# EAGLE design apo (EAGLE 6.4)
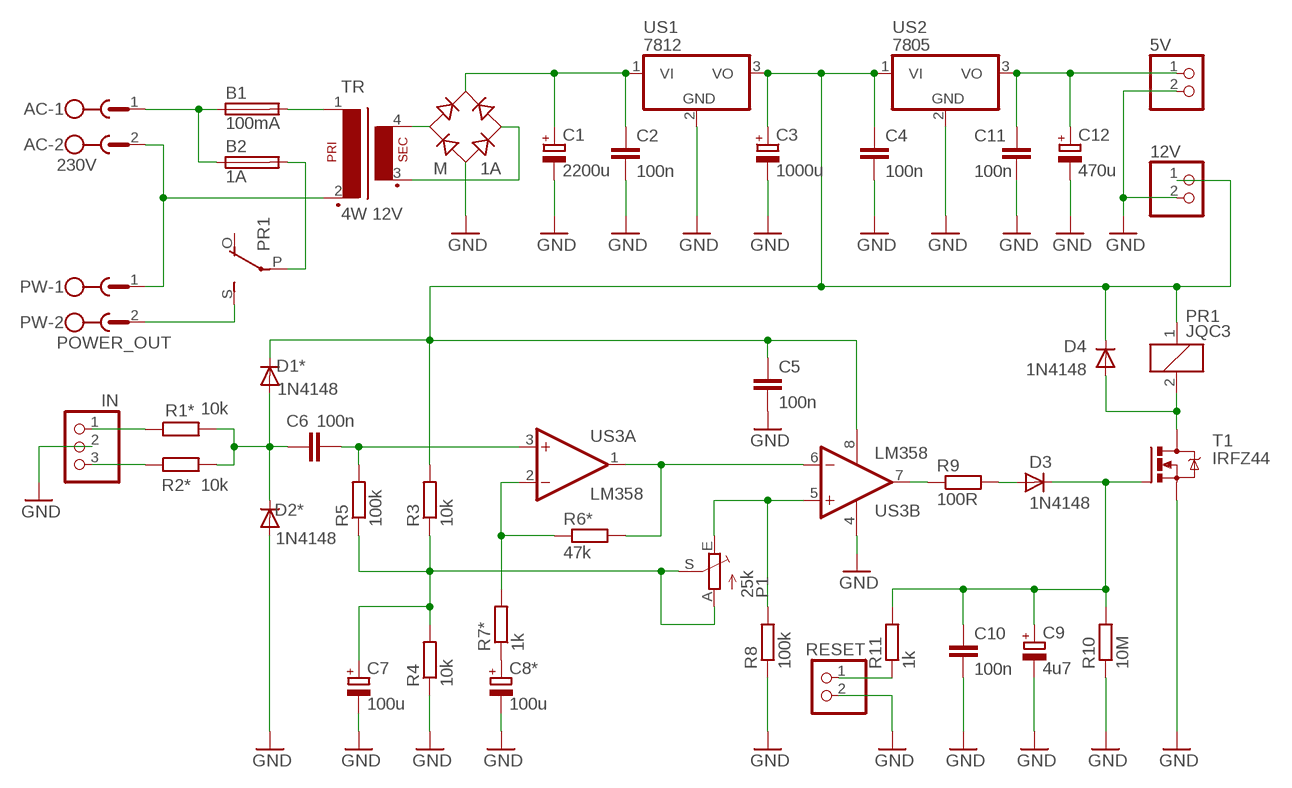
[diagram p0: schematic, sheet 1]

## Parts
5V  PINHD-1X2  [1X02]
12V  PINHD-1X2  [1X02]
AC  230V  MSTBV2  [MSTBV2]
B1  100mA  SH22,5A  [SH22,5A]
B2  1A  SH22,5A  [SH22,5A]
C1  2200u  CPOL-EUE5-13  [E5-13]
C2  100n  C-EU050-025X075  [C050-025X075]
C3  1000u  CPOL-EUE5-10.5  [E5-10,5]
C4  100n  C-EU050-025X075  [C050-025X075]
C5  100n  C-EU050-025X075  [C050-025X075]
C6  100n  C-EU050-025X075  [C050-025X075]
C7  100u  CPOL-EUE2.5-7  [E2,5-7]
C8*  100u  CPOL-EUE2.5-7  [E2,5-7]
C9  4u7  CPOL-EUE5-8.5  [E5-8,5]
C10  100n  C-EU050-025X075  [C050-025X075]
C11  100n  C-EU050-025X075  [C050-025X075]
C12  470u  CPOL-EUE5-8.5  [E5-8,5]
D1*  1N4148  1N4148DO35-7  [DO35-7]
D2*  1N4148  1N4148DO35-7  [DO35-7]
D3  1N4148  1N4148DO35-7  [DO35-7]
D4  1N4148  1N4148DO35-7  [DO35-7]
IN  PINHD-1X3  [1X03]
M  1A  RB1A  [RB1A]
P1  25k  TRIM_EU-RS3  [RS3]
PR1  JQC3  G5L  [G5LE]
PW  POWER_OUT  MSTBV2  [MSTBV2]
R1*  10k  R-EU_0207/10  [0207/10]
R2*  10k  R-EU_0207/10  [0207/10]
R3  10k  R-EU_0207/10  [0207/10]
R4  10k  R-EU_0207/10  [0207/10]
R5  100k  R-EU_0207/10  [0207/10]
R6*  47k  R-EU_0207/10  [0207/10]
R7*  1k  R-EU_0207/10  [0207/10]
R8  100k  R-EU_0207/10  [0207/10]
R9  100R  R-EU_0207/10  [0207/10]
R10  10M  R-EU_0207/10  [0207/10]
R11  1k  R-EU_0207/10  [0207/10]
RESET  PINHD-1X2  [1X02]
T1  IRFZ44  IRF540  [TO220BV]
TR  4W 12V  VP31  [VP31]
US1  7812  7812TV  [TO220V]
US2  7805  7805TV  [TO220V]
US3  LM358  LM358N  [DIL08]

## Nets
GND: 5V.2 12V.2 C1.- C2.2 C3.- C4.2 C5.2 C7.- C8*.- C9.- C10.2 C11.2 C12.- D2*.A IN.2 M.- R4.1 R8.1 R10.1 RESET.2 T1.S US1.2(GND) US2.2(GND) US3.4(P:V-)
N$1: AC.2 PW.1 TR.2
N$2: AC.1 B1.1 B2.1
N$3: B1.2 TR.1
N$4: M.AC1 TR.4(S4)
N$5: B2.2 PR1.P(2:P)
N$6: PR1.S(2:S) PW.2
N$7: M.AC2 TR.3(S3)
N$8: C1.+ C2.1 M.+ US1.1(VI)
N$9: 12V.1 C3.+ C4.1 C5.1 D1*.C D4.C PR1.1 R3.2 US1.3(VO) US2.1(VI) US3.8(P:V+)
N$10: IN.1 R1*.1
N$11: C6.2 R5.2 US3.3(A:+IN)
N$12: IN.3 R2*.1
N$13: R6*.1 R7*.2 US3.2(A:-IN)
N$14: C6.1 D1*.A D2*.C R1*.2 R2*.2
N$15: C8*.+ R7*.1
N$16: R6*.2 US3.1(A:OUT) US3.6(B:-IN)
N$17: C7.+ P1.A P1.S R3.1 R4.2 R5.1
N$18: D4.A PR1.2 T1.D
N$19: P1.E R8.2 US3.5(B:+IN)
N$21: C9.+ C10.1 D3.C R10.2 R11.2 T1.G
N$22: R9.1 US3.7(B:OUT)
N$23: D3.A R9.2
N$25: R11.1 RESET.1
N$26: 5V.1 C11.1 C12.+ US2.3(VO)
Unconnected: PR1.O(2:O)

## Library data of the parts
5V 12V RESET = pinhead:PINHD-1X2: PIN HEADER
AC PW = con-phoenix-508:MSTBV2: PHOENIX
B1 B2 = fuse:SH22,5A: FUSE HOLDER
C1 C3 C7 C8* C9 C12 = rcl:CPOL-EU: POLARIZED CAPACITOR, European symbol
C2 C4-C6 C10 C11 = rcl:C-EU: CAPACITOR, European symbol
D1* D2* D3 D4 = diode:1N4148: DIODE
IN = pinhead:PINHD-1X3: PIN HEADER
M = rectifier:RB1A: RECTIFIER 1 A
P1 = pot:TRIM_EU-: POTENTIOMETER
PR1 = relay:G5L: RELAY 1 x switch, 10 A/120 V AC, 8 A/30 V ADC, Omron
R1* R2* R3-R5 R6* R7* R8-R11 = rcl:R-EU_: RESISTOR, European symbol
T1 = transistor-power:IRF540: HEXFET Power MOSFET
TR = trafo:VP31: TRANSFORMER 1 primary winding, 1 secondary winding BLOCK
US1 US2 = linear:78*: Positive VOLTAGE REGULATOR Source: http://cache.national.com/ds/LM/LM78L05.pdf http://www.fairchildsemi.com/ds/LM/LM7805.pdf
US3 = linear:LM358: OP AMP also LM158; LM258; LM2904 Source: http://cache.national.com/ds/LM/LM158.pdf

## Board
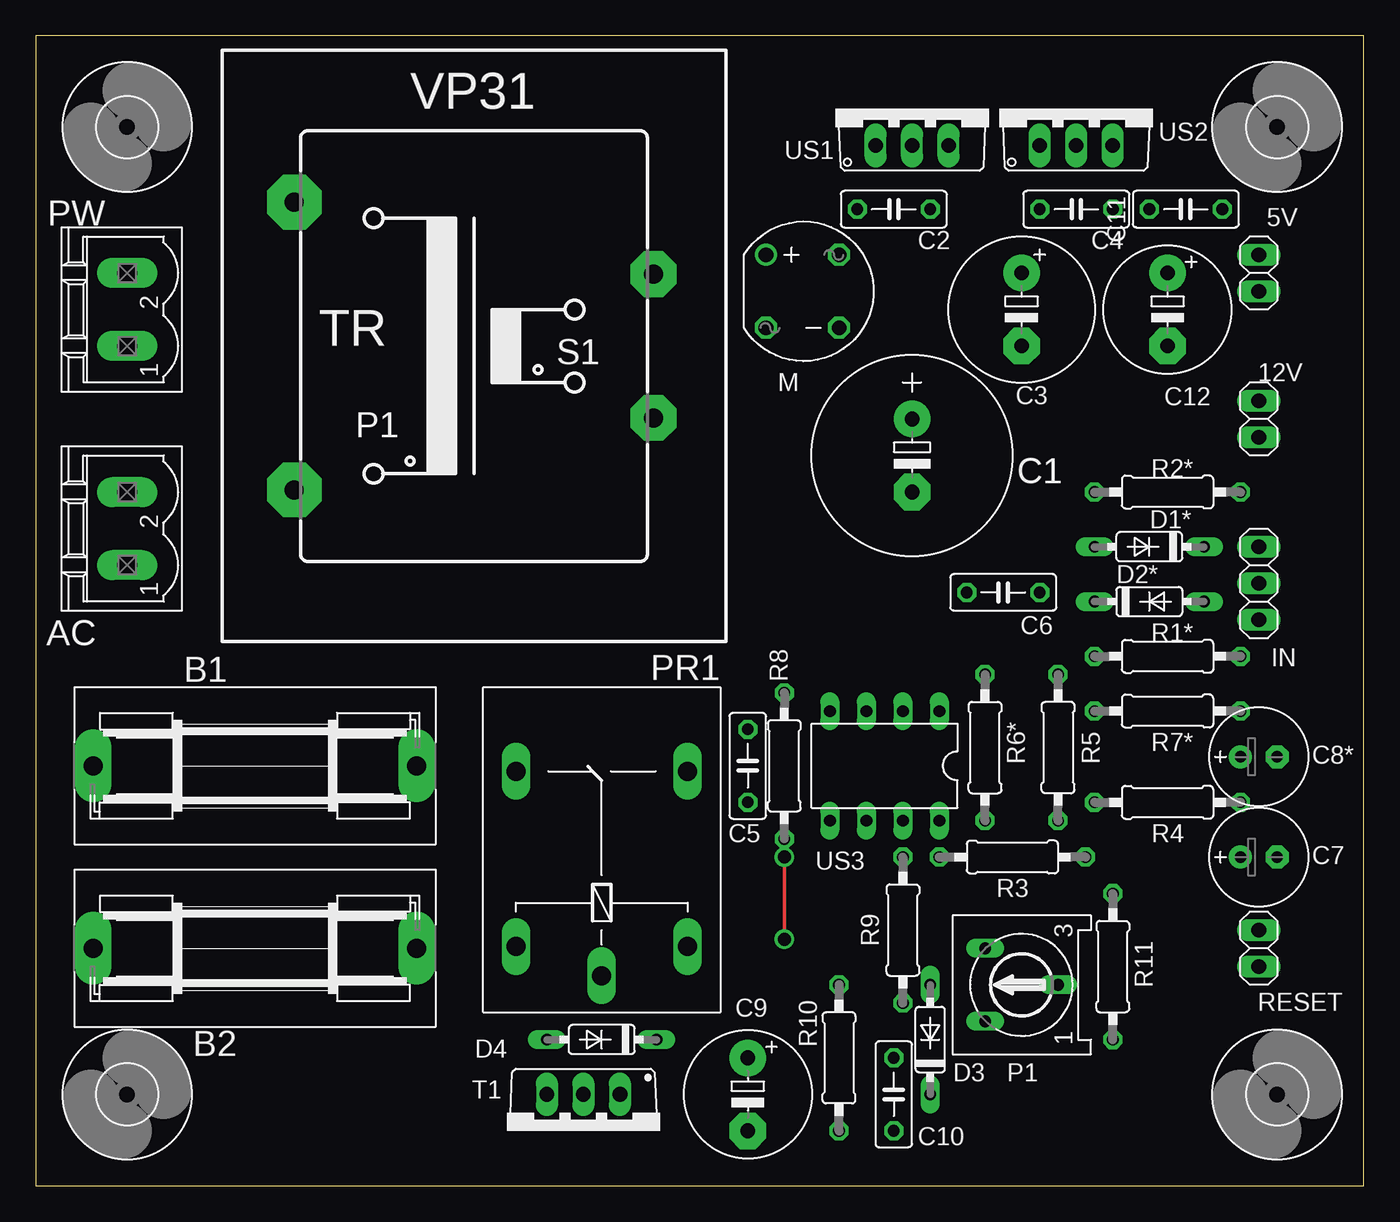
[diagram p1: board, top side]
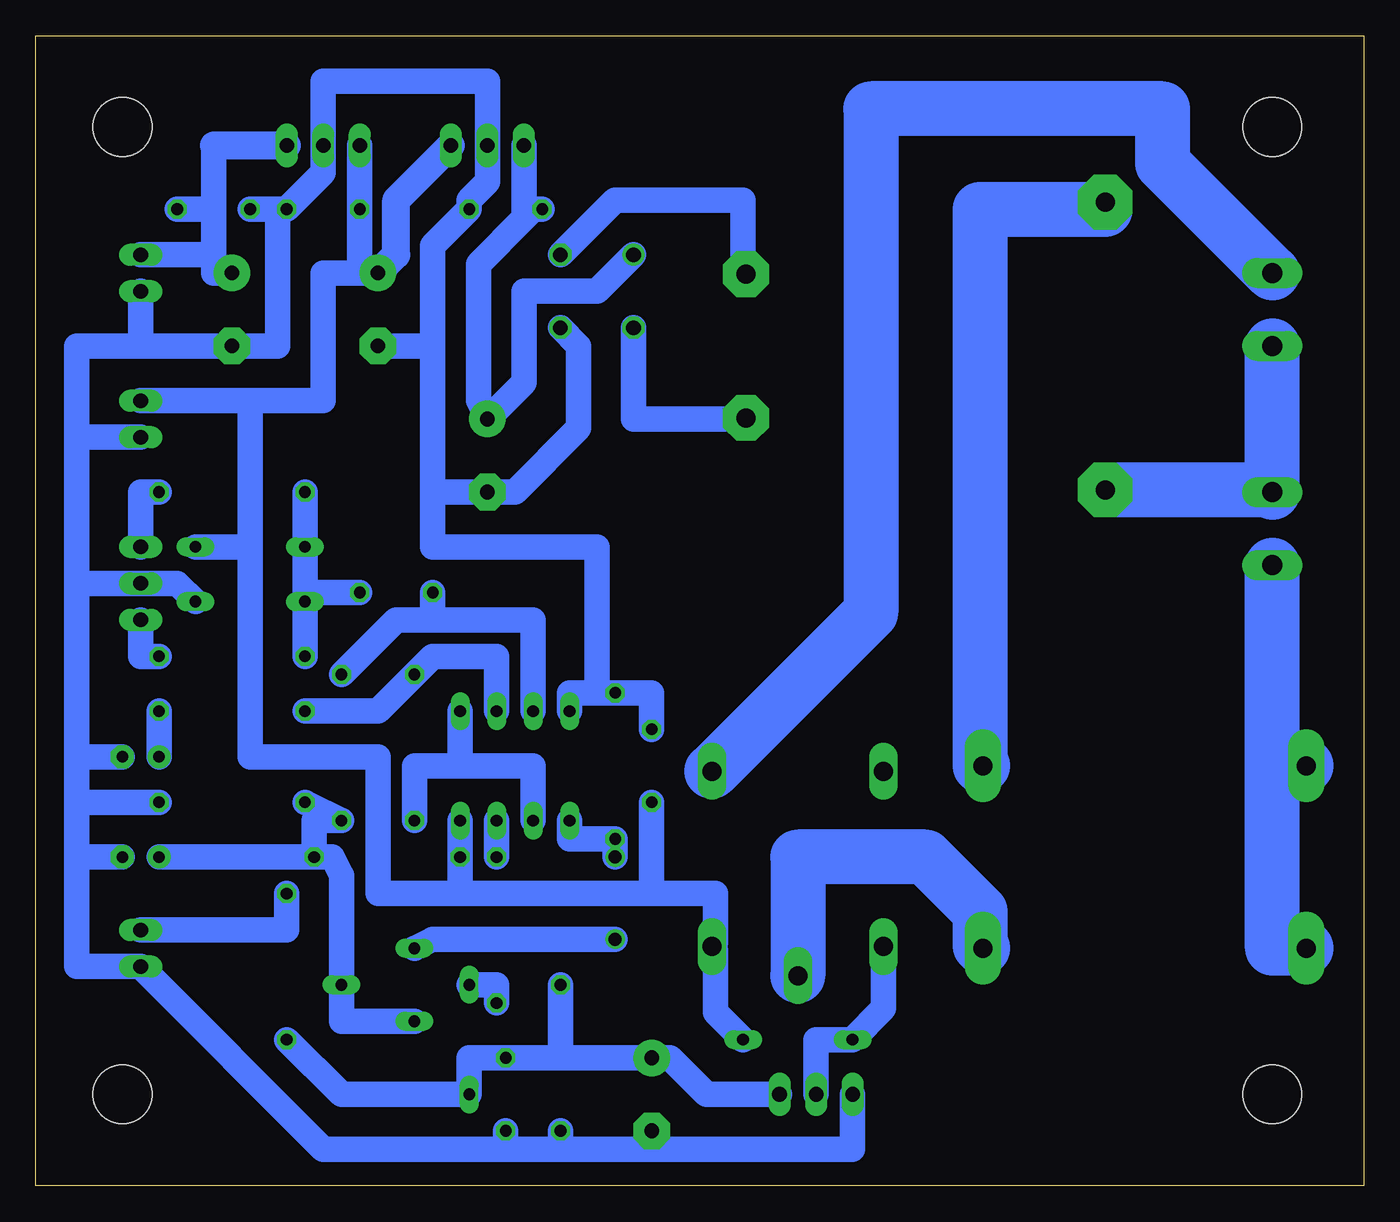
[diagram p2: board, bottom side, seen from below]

Size 92.38 x 80 mm. Coordinates in mm from the lower left corner, seen from the top.
Outline: 0,0 92.38,0 92.38,80 0,80 0,0
Copper layers (1*16): Top 0.035mm / dielectric 1.5mm / Bottom 0.035mm
Design rules "default": minimum track width 10mil, minimum drill 24mil, track to track 8mil, track to pad 8mil, pad to pad 8mil, via to via 8mil, smd to smd 8mil, copper to edge 40mil, drill to drill 8mil, minimum pad ring 10mil, minimum via ring 8mil, stop-mask expansion 4mil, vias tented up to drill 0mil, thermal gap 10mil

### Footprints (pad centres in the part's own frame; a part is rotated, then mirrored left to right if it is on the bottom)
1X02 = drill 1.016 long: 1 -1.27,0; 2 1.27,0
MSTBV2 = drill 1.397 long: 1 -2.54,0; 2 2.54,0
SH22,5A = drill 1.321 pad 2.54 long: 1 -11.252,0; 2 11.252,0
E5-13 = drill 1.016 pad 2.54: + -2.54,0 | drill 1.016 pad 2.54 octagon: - 2.54,0
C050-025X075 = drill 0.813 octagon: 1 -2.54,0; 2 2.54,0
E5-10,5 = drill 1.016 pad 2.54: + -2.54,0 | drill 1.016 pad 2.54 octagon: - 2.54,0
E2,5-7 = drill 0.813 pad 1.6: + -1.27,0 | drill 0.813 pad 1.6 octagon: - 1.27,0
E5-8,5 = drill 1.016 pad 2.54: + -2.54,0 | drill 1.016 pad 2.54 octagon: - 2.54,0
DO35-7 = drill 0.813 long: A 3.81,0; C -3.81,0
1X03 = drill 1.016 long: 1 -2.54,0; 2 0,0; 3 2.54,0
RB1A = drill 1.016: + -2.54,2.54 | drill 1.016 octagon: - 2.54,-2.54; AC1 2.54,2.54; AC2 -2.54,-2.54
RS3 = drill 0.813 long: A -2.54,2.54; E 2.54,2.54; S 0,-2.54
G5LE = drill 1.321 long: 1 -7.493,-5.969; 2 -7.493,5.969; O 4.699,5.969; P -9.525,0; S 4.699,-5.969
0207/10 = drill 0.813 octagon: 1 -5.08,0; 2 5.08,0
TO220BV = drill 1.016 long: D 0,-2.54; G -2.54,-2.54; S 2.54,-2.54
VP31 = drill 1.321 pad 3.81 octagon: 1 -12.497,10.008; 2 -12.497,-10.008 | drill 1.321 pad 3.175 octagon: 3 12.497,-5.004; 4 12.497,5.004
4,1 = hole 4.1: 0,0
TO220V = drill 1.016 long: 1 -2.54,-2.54; 2 0,-2.54; 3 2.54,-2.54
DIL08 = drill 0.813 long: 1 -3.81,-3.81; 2 -1.27,-3.81; 3 1.27,-3.81; 4 3.81,-3.81; 5 3.81,3.81; 6 1.27,3.81; 7 -1.27,3.81; 8 -3.81,3.81

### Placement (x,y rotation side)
5V  85.09,63.5 270 top
12V  85.09,53.34 270 top
AC  6.35,45.72 90 top
B1  15.24,29.21 0 top
B2  15.24,16.51 0 top
C1  60.96,50.8 270 top
C2  59.69,67.94 0 top
C3  68.58,60.96 270 top
C4  72.39,67.94 0 top
C5  49.53,29.21 90 top
C6  67.31,41.27 180 top
C7  85.09,22.86 0 top
C8*  85.09,29.84 0 top
C9  49.53,6.35 270 top
C10  59.69,6.35 270 top
C11  80.01,67.94 180 top
C12  78.74,60.96 270 top
D1*  77.47,44.45 180 top
D2*  77.47,40.64 0 top
D3  62.23,10.16 90 top
D4  39.37,10.16 180 top
IN  85.09,41.91 90 top
M  53.34,62.23 0 top
P1  68.58,13.97 90 top
PR1  39.37,24.13 90 top
PW  6.35,60.96 90 top
R1*  78.74,36.83 180 top
R2*  78.74,48.26 180 top
R3  67.94,22.86 180 top
R4  78.74,26.67 180 top
R5  71.12,30.48 90 top
R6*  66.04,30.48 270 top
R7*  78.74,33.02 180 top
R8  52.07,29.21 270 top
R9  60.33,17.78 270 top
R10  55.88,8.89 90 top
R11  74.93,15.24 270 top
RESET  85.09,16.51 270 top
T1  38.1,3.81 180 top
TR  30.48,58.42 0 top
U$1  [4,1]  6.35,73.66 0 top
U$2  [4,1]  6.35,6.35 0 top
U$3  [4,1]  86.36,6.35 0 top
U$4  [4,1]  86.36,73.66 0 top
US1  60.96,74.93 0 top
US2  72.39,74.93 0 top
US3  59.05,29.21 180 top

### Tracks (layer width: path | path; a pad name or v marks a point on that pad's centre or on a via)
GND
  Bottom 1.778: T1.S 35.56,2.54 49.53,2.54 | 49.53,2.54 C9.- | 49.53,2.54 55.88,2.54 | 55.88,2.54 R10.1 | 55.88,2.54 59.69,2.54 | 59.69,2.54 C10.2 | 59.69,2.54 72.39,2.54 RESET.2 89.53,15.24 89.53,22.86 | 89.53,22.86 89.53,26.67 | 89.53,26.67 89.53,29.84 | 89.53,29.84 89.53,41.91 | 89.53,41.91 IN.2 82.55,41.91 D2*.A | 89.53,29.84 C8*.- | US3.4 55.24,34.29 53.34,34.29 | 89.53,22.86 C7.- | 89.53,26.67 R4.1 | M.- 54.61,58.42 54.61,52.7 59.05,48.26 C1.- 64.77,48.26 | 64.77,58.42 64.77,48.26 | 64.77,58.42 C3.- | 64.77,58.42 64.77,65.41 C2.2 62.23,68.58 60.96,69.85 US1.2 60.96,76.83 72.39,76.83 US2.2 72.39,70.48 C4.2 75.56,67.94 | C5.2 49.53,34.29 R8.1 53.34,34.29 | 53.34,34.29 53.34,44.45 64.77,44.45 64.77,48.26 | 89.53,41.91 89.53,52.07 | 89.53,52.07 89.53,58.42 85.09,58.42 | 85.09,58.42 C12.- 75.56,58.42 75.56,67.94 | 85.09,58.42 5V.2 | 89.53,52.07 12V.2 | 75.56,67.94 C11.2
N$1
  Bottom 2.54: AC.2 6.35,48.41
  Bottom 3.81: AC.2 PW.1 | 6.35,48.41 TR.2
N$2
  Bottom 3.81: 6.35,29.21 AC.1 | 6.35,29.21 B1.1 | B2.1 6.35,16.51 6.35,29.21
N$3
  Bottom 3.81: B1.2 26.67,29.21 26.67,67.94 17.98,67.94 TR.1
N$4
  Bottom 1.778: M.AC1 52.07,68.58 43.18,68.58 43.18,63.63 TR.4
N$5
  Bottom 3.81: PR1.P 39.37,22.86 30.48,22.86 26.67,19.05 26.67,16.69 B2.2
N$6
  Bottom 3.81: PW.2 12.7,69.85 13.97,71.12 13.97,74.93 34.29,74.93 34.29,39.88 PR1.S
N$7
  Bottom 1.778: M.AC2 50.8,53.34 43.05,53.34 TR.3
N$8
  Bottom 1.778: M.+ 53.34,62.23 58.42,62.23 58.42,55.88 C1.+ 61.59,54.61 61.59,64.14 58.42,67.31 | 58.42,67.31 US1.1 | C2.1 57.78,67.94 58.42,67.31
N$9
  Bottom 1.778: D4.C 45.09,12.06 45.09,16.38 PR1.1 45.09,16.89 45.09,20.32 49.53,20.32 | 77.47,44.45 77.47,54.61 | 77.47,54.61 72.39,54.61 72.39,63.5 69.85,63.5 | 69.85,63.5 C3.+ | 77.47,44.45 D1*.C | US3.8 R3.2 62.87,20.32 | 49.53,20.32 62.87,20.32 | 77.47,44.45 77.47,29.84 68.58,29.84 68.58,20.32 62.87,20.32 | 49.53,20.32 C5.1 | US2.1 C4.1 69.85,63.5 | 77.47,54.61 12V.1
  Bottom 1.93: C3.+ 67.31,64.77 67.31,68.58 US1.3
N$10
  Bottom 1.778: R1*.1 85.09,36.83 IN.1
N$11
  Bottom 1.778: US3.3 57.78,39.37 64.77,39.37 | 64.77,39.37 67.31,39.37 R5.2 | 64.77,39.37 C6.2
N$12
  Bottom 1.778: IN.3 85.09,48.26 R2*.1
N$13
  Bottom 1.778: US3.2 60.33,36.83 64.77,36.83 R6*.1 68.58,33.02 R7*.2
N$14
  Bottom 1.778: R2*.2 D1*.A 73.66,41.27 | R1*.2 D2*.C 73.66,41.27 | C6.1 73.66,41.27
N$15
  Bottom 1.778: C8*.+ R7*.1
N$16
  Bottom 1.778: US3.6 57.78,29.21 62.87,29.21 | 62.87,29.21 US3.1 | 62.87,29.21 66.04,29.21 R6*.2
N$17
  Bottom 1.778: R3.1 73.03,25.4 R5.1 R4.2 | P1.A 71.12,11.43 P1.S 71.12,21.59 71.75,22.86 R3.1 | R3.1 C7.+
N$18
  Bottom 1.778: PR1.2 33.4,12.32 D4.A 38.1,10.16 T1.D
N$19  (via drill 0.9)
  Top 0.254: v52.07,17.14 v52.07,22.86
  Bottom 1.778: US3.5 55.24,24.13 R8.2 v52.07,22.86 | v52.07,17.14 64.77,17.14 P1.E
N$21
  Bottom 1.778: T1.G 45.72,6.35 48.26,8.89 C9.+ 55.88,8.89 | 55.88,8.89 C10.1 62.23,8.89 D3.C 71.12,6.35 R11.2 | 55.88,8.89 R10.2
N$22
  Bottom 1.778: R9.1 US3.7
N$23
  Bottom 1.778: R9.2 60.33,13.97 D3.A
N$25
  Bottom 1.778: RESET.1 74.93,17.78 R11.1
N$26
  Bottom 1.778: 80.01,72.39 80.01,67.94 | 80.01,67.94 80.01,64.77 | 80.01,64.77 80.01,63.5 C12.+ | C11.1 80.01,67.94 | 5V.1 80.01,64.77
  Bottom 1.93: 80.01,72.39 US2.3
